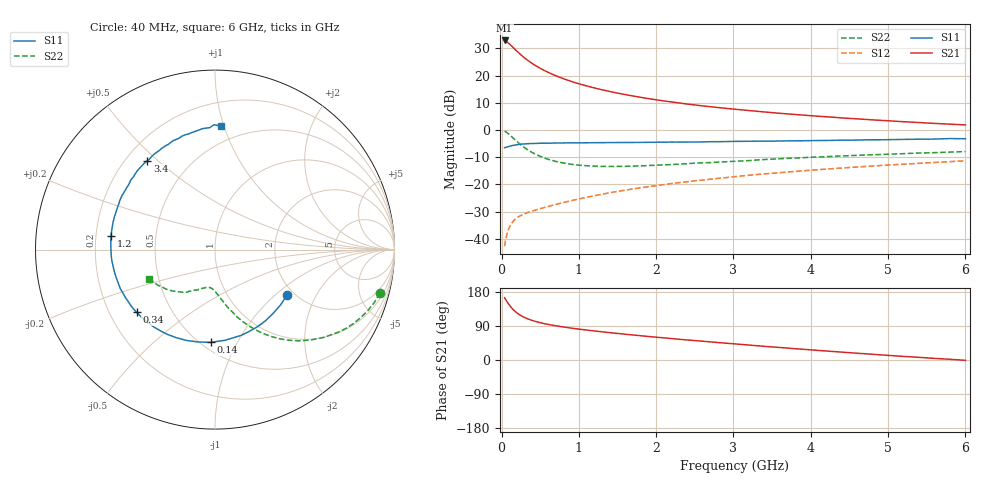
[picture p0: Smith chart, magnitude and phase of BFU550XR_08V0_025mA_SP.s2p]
! Filename:  P:\Prog\Test\Noise\ATS_data\Testdata_Net\03 Spar\BFU550XR_APG2013_45_C05_08p0V_025mA_SP_CM01_D.s2p
! Date/Time: Tue 06/Aug/2013 14:38:17
! BFU550XR_APG2013_45_C05_08p0V_25to35mA_SP_CM01_Bias1_R.s2p
! MDIF S-parameter v. bias file
! BFU550XR_APG2013_45_C05_08p0V_25to35mA_SP_CM01
! Date/time Mon Aug 05 17:22:52 2013
! bias mode 1
! bias variable = I_out
! VAR bias_var= 1
! VAR V_out= 8.0000
! VAR I_out= 25.0000
! VAR V_in= 0.8077
! VAR I_in= 0.2654
! Device data file deembeded for feedlines and parallel
! Original file: \03 Spar\BFU550XR_APG2013_45_C05_08p0V_025mA_SP_CM01_R.s2p
! Feed-files: PR006V01_02082013_Feed1.s2p, PR006V01_02082013_Feed2.s2p
! Parallel-file: PR006V01_02082013_Par.s2p
# MHz S MA R 50
!  Freq-MHz  S11-mag  S11-arg  S21-mag  S21-arg  S12-mag  S12-arg  S22-mag  S22-arg
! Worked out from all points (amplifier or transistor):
!   98 points, 40 MHz to 6 GHz, reference 50 ohm
!   highest |S21| = 32.9 dB at 40 MHz (marker M1)
!   |S21| within 3 dB of that: start of sweep to 164.4 MHz
!   unconditionally stable (mu >= 1): 1.43 GHz to 3.185 GHz
!   at 300 MHz: K = 0.49, MSG = 28.6 dB, |S12| = -30.8 dB
!   at 1.6 GHz: K = 1.01, MAG = 16.9 dB, |S12| = -22.1 dB
!   at 6 GHz: K = 0.87, MSG = 6.6 dB, |S12| = -11.4 dB
!   S11 on the Smith chart (normalised r, x): 40 MHz: 1.83, -1.20; 140 MHz: 0.56, -0.78; 340 MHz: 0.31, -0.32; 1.2 GHz: 0.26, +0.06; 3.4 GHz: 0.29, +0.46; 6 GHz: 0.37, +0.98
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40  0.474 -32.5  44.29 164.3  0.007302 78.8  0.9496 -14.7
50  0.478 -40.1  43.29 160.3  0.009017 75.5  0.9354 -18.4
70  0.4862 -54.5  41.59 154.3  0.01216 71.2  0.8963 -25.0
90  0.494 -67.3  39.44 148.1  0.01486 67.0  0.8508 -31.1
120  0.5084 -83.7  36.18 140.0  0.01819 61.8  0.7791 -38.9
140  0.5174 -92.7  33.98 135.4  0.02005 59.1  0.7328 -43.4
180  0.5308 -107.7  29.84 127.6  0.02309 54.9  0.6487 -51.0
220  0.5418 -119.3  26.43 121.2  0.02535 52.3  0.5778 -56.9
280  0.5526 -132.1  22.24 114.0  0.02804 50.4  0.4936 -63.7
340  0.5594 -141.4  19.06 108.6  0.03028 49.6  0.4315 -68.7
440  0.5662 -152.5  15.29 101.8  0.03373 50.3  0.358 -74.7
600  0.5721 -164.3  11.54 94.1  0.03912 52.3  0.2904 -81.4
800  0.578 -174.0  8.792 87.2  0.04627 54.9  0.248 -87.2
1050  0.581 177.0  6.758 80.3  0.05589 57.4  0.2226 -92.3
1200  0.5841 172.6  5.936 76.7  0.06187 58.2  0.2165 -95.1
1600  0.5891 162.4  4.479 68.0  0.07822 59.0  0.2143 -101.5
2050  0.5968 152.9  3.505 59.3  0.09679 58.5  0.2273 -107.8
3100  0.6179 132.7  2.35 41.1  0.1425 54.2  0.2687 -120.7
3400  0.6221 127.2  2.146 36.0  0.1558 52.1  0.2862 -123.8
4100  0.6403 115.6  1.787 25.2  0.1863 47.5  0.3186 -132.7
5200  0.6708 98.2  1.418 9.5  0.2351 39.0  0.3671 -146.1
6000  0.6891 87.0  1.24 -1.0  0.2706 32.0  0.4014 -156.1
